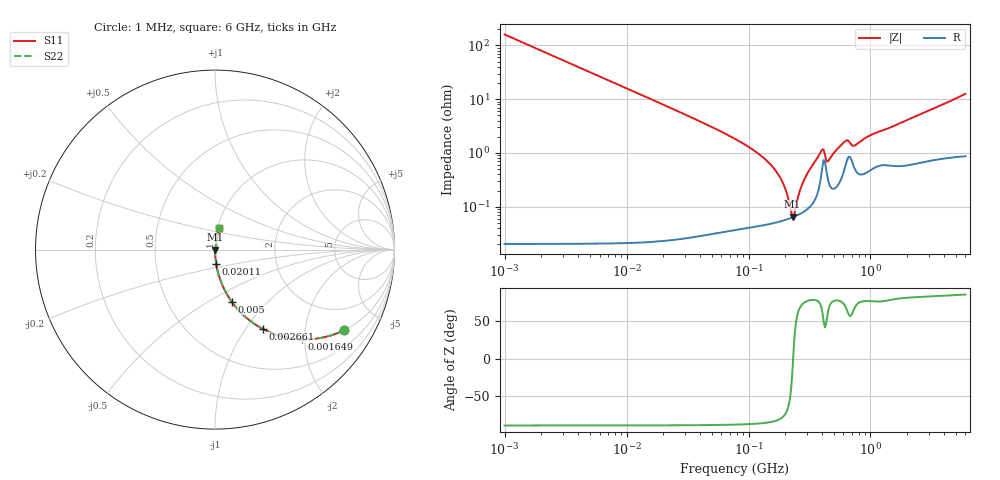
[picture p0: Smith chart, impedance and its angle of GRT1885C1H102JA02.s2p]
!Murata Part Number: GRT1885C1H102JA02
!These Parameters are Measured in Series Mode Connection
!Data Generated on Jun 19, 2026
!  o--ll--o
!Port1  Port2
!  o------o
!Operation Temp=25[degC], DC Bias Voltage=0[V]
!Freq. Start=1000[kHz] Stop=6[GHz] 401[Steps]
# Hz S RI R 50
!Freq.(Hz) S11(Real) S11(Imag) S21(Real) S21(Imag) S12(Real) S12(Imag) S22(Real) S22(Imag)
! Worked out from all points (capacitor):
!   401 points, 1 MHz to 6 GHz, reference 50 ohm
!   read as one part in series: C = 996 pF near 1.044 MHz
!   lowest |Z| = 65.3 mohm at 229.8 MHz (marker M1)
!   series resonance near 232.1 MHz, so ESL is about 470 pH
!   S11 on the Smith chart (normalised r, x): 1 MHz: 1.00, -3.20; 1.649 MHz: 1.00, -1.94; 2.661 MHz: 1.00, -1.20; 5 MHz: 1.00, -0.64; 20.11 MHz: 1.00, -0.16; 6 GHz: 1.02, +0.25
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1000000  0.7187 -0.4496  0.2813 0.4496  0.2813 0.4496  0.7187 -0.4496
1649087  0.4844 -0.4997  0.5156 0.4997  0.5156 0.4997  0.4844 -0.4997
2660982  0.2652 -0.4413  0.7348 0.4413  0.7348 0.4413  0.2652 -0.4413
4293785  0.1218 -0.3268  0.8782 0.3268  0.8782 0.3268  0.1218 -0.3268
4999862  0.0928 -0.2898  0.9072 0.2898  0.9072 0.2898  0.0928 -0.2898
1.843659e7  0.00758 -0.0854  0.9924 0.0854  0.9924 0.0854  0.00758 -0.0854
2.011232e7  0.0064 -0.0783  0.9936 0.0783  0.9936 0.0783  0.0064 -0.0783
7.745967e7  0.000704 -0.0183  0.9993 0.0183  0.9993 0.0183  0.000704 -0.0183
1.223006e8  0.000528 -0.00946  0.9995 0.00946  0.9995 0.00946  0.000528 -0.00946
1.622626e8  0.000527 -0.00508  0.9995 0.00508  0.9995 0.00508  0.000527 -0.00508
1.930997e8  0.000563 -0.00259  0.9994 0.00259  0.9994 0.00259  0.000563 -0.00259
2.297971e8  0.000638 -0.00014  0.9994 0.00014  0.9994 0.00014  0.000638 -0.00014
2.400133e8  0.000665 0.000479  0.9993 -0.000479  0.9993 -0.000479  0.000665 0.000479
2.794814e8  0.0008 0.00273  0.9992 -0.00273  0.9992 -0.00273  0.0008 0.00273
3.325952e8  0.00115 0.00569  0.9988 -0.00569  0.9988 -0.00569  0.00115 0.00569
3.958029e8  0.00413 0.0102  0.9959 -0.0102  0.9959 -0.0102  0.00413 0.0102
4.509737e8  0.00305 0.00645  0.9969 -0.00645  0.9969 -0.00645  0.00305 0.00645
6.249308e8  0.00615 0.0155  0.9939 -0.0155  0.9939 -0.0155  0.00615 0.0155
7.436952e8  0.0052 0.0128  0.9948 -0.0128  0.9948 -0.0128  0.0052 0.0128
9.866994e8  0.00509 0.0205  0.9949 -0.0205  0.9949 -0.0205  0.00509 0.0205
1.428092e9  0.00663 0.0285  0.9934 -0.0285  0.9934 -0.0285  0.00663 0.0285
6e9  0.0238 0.1219  0.9762 -0.1219  0.9762 -0.1219  0.0238 0.1219
